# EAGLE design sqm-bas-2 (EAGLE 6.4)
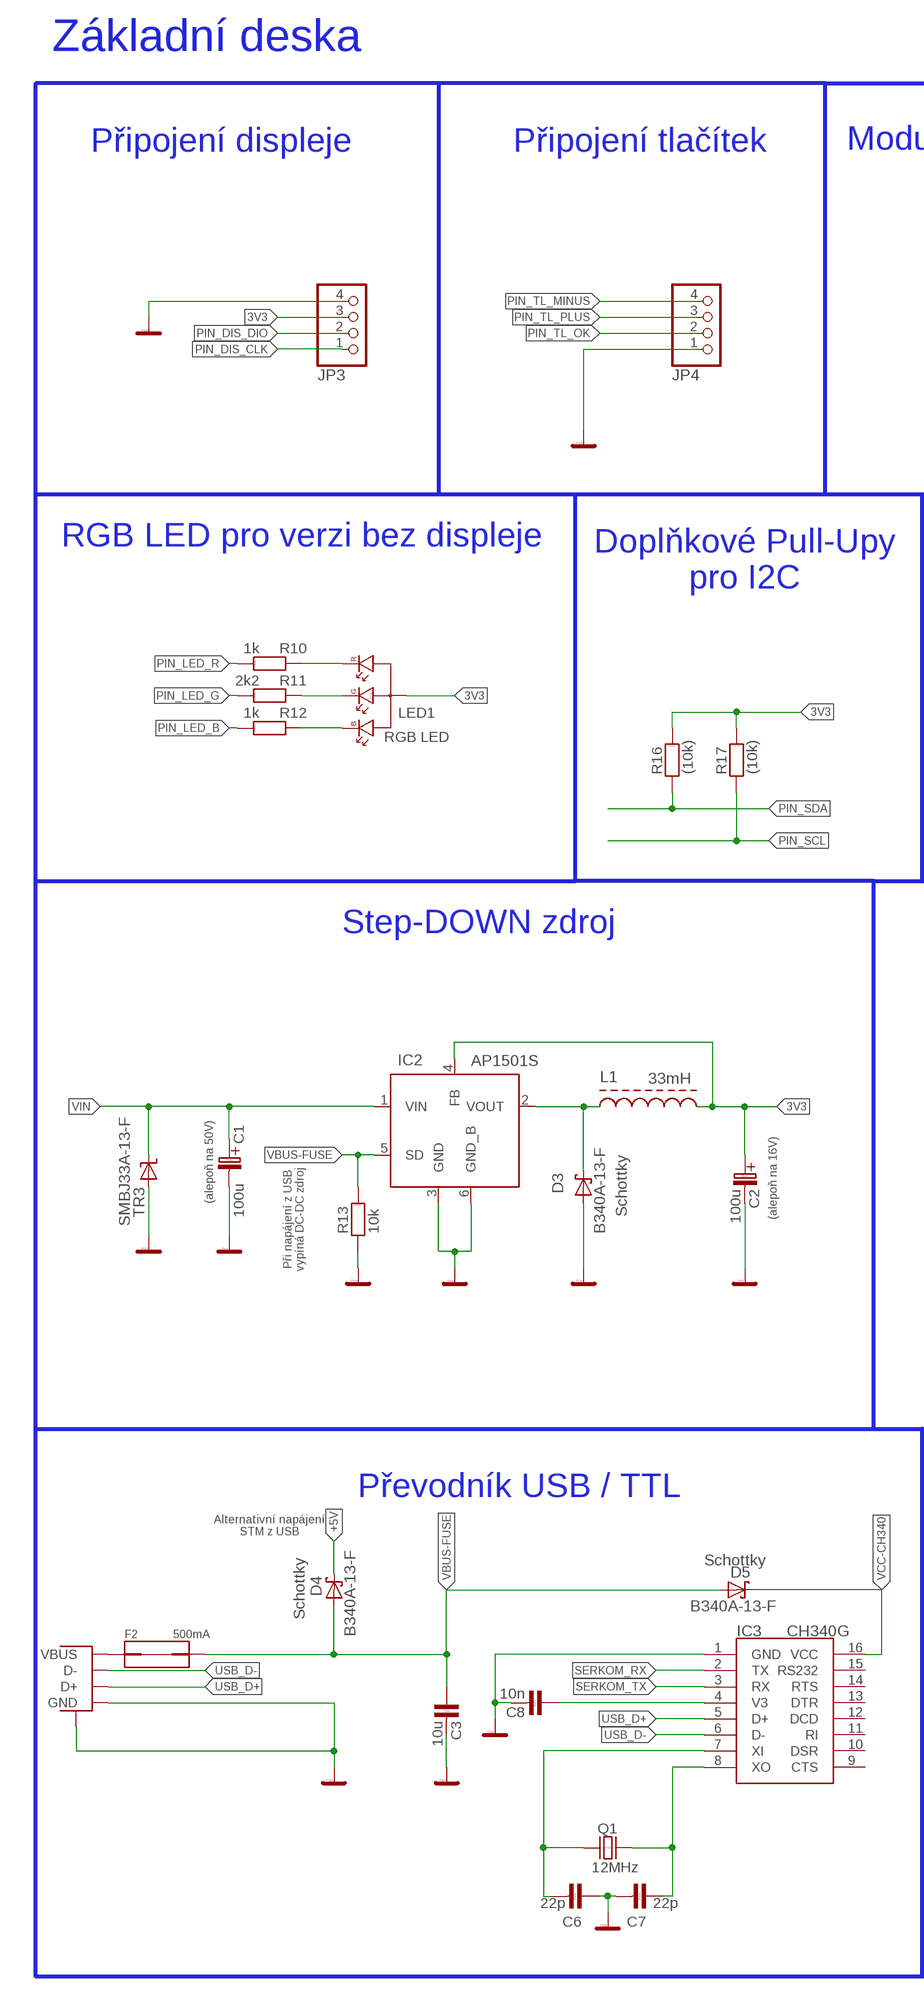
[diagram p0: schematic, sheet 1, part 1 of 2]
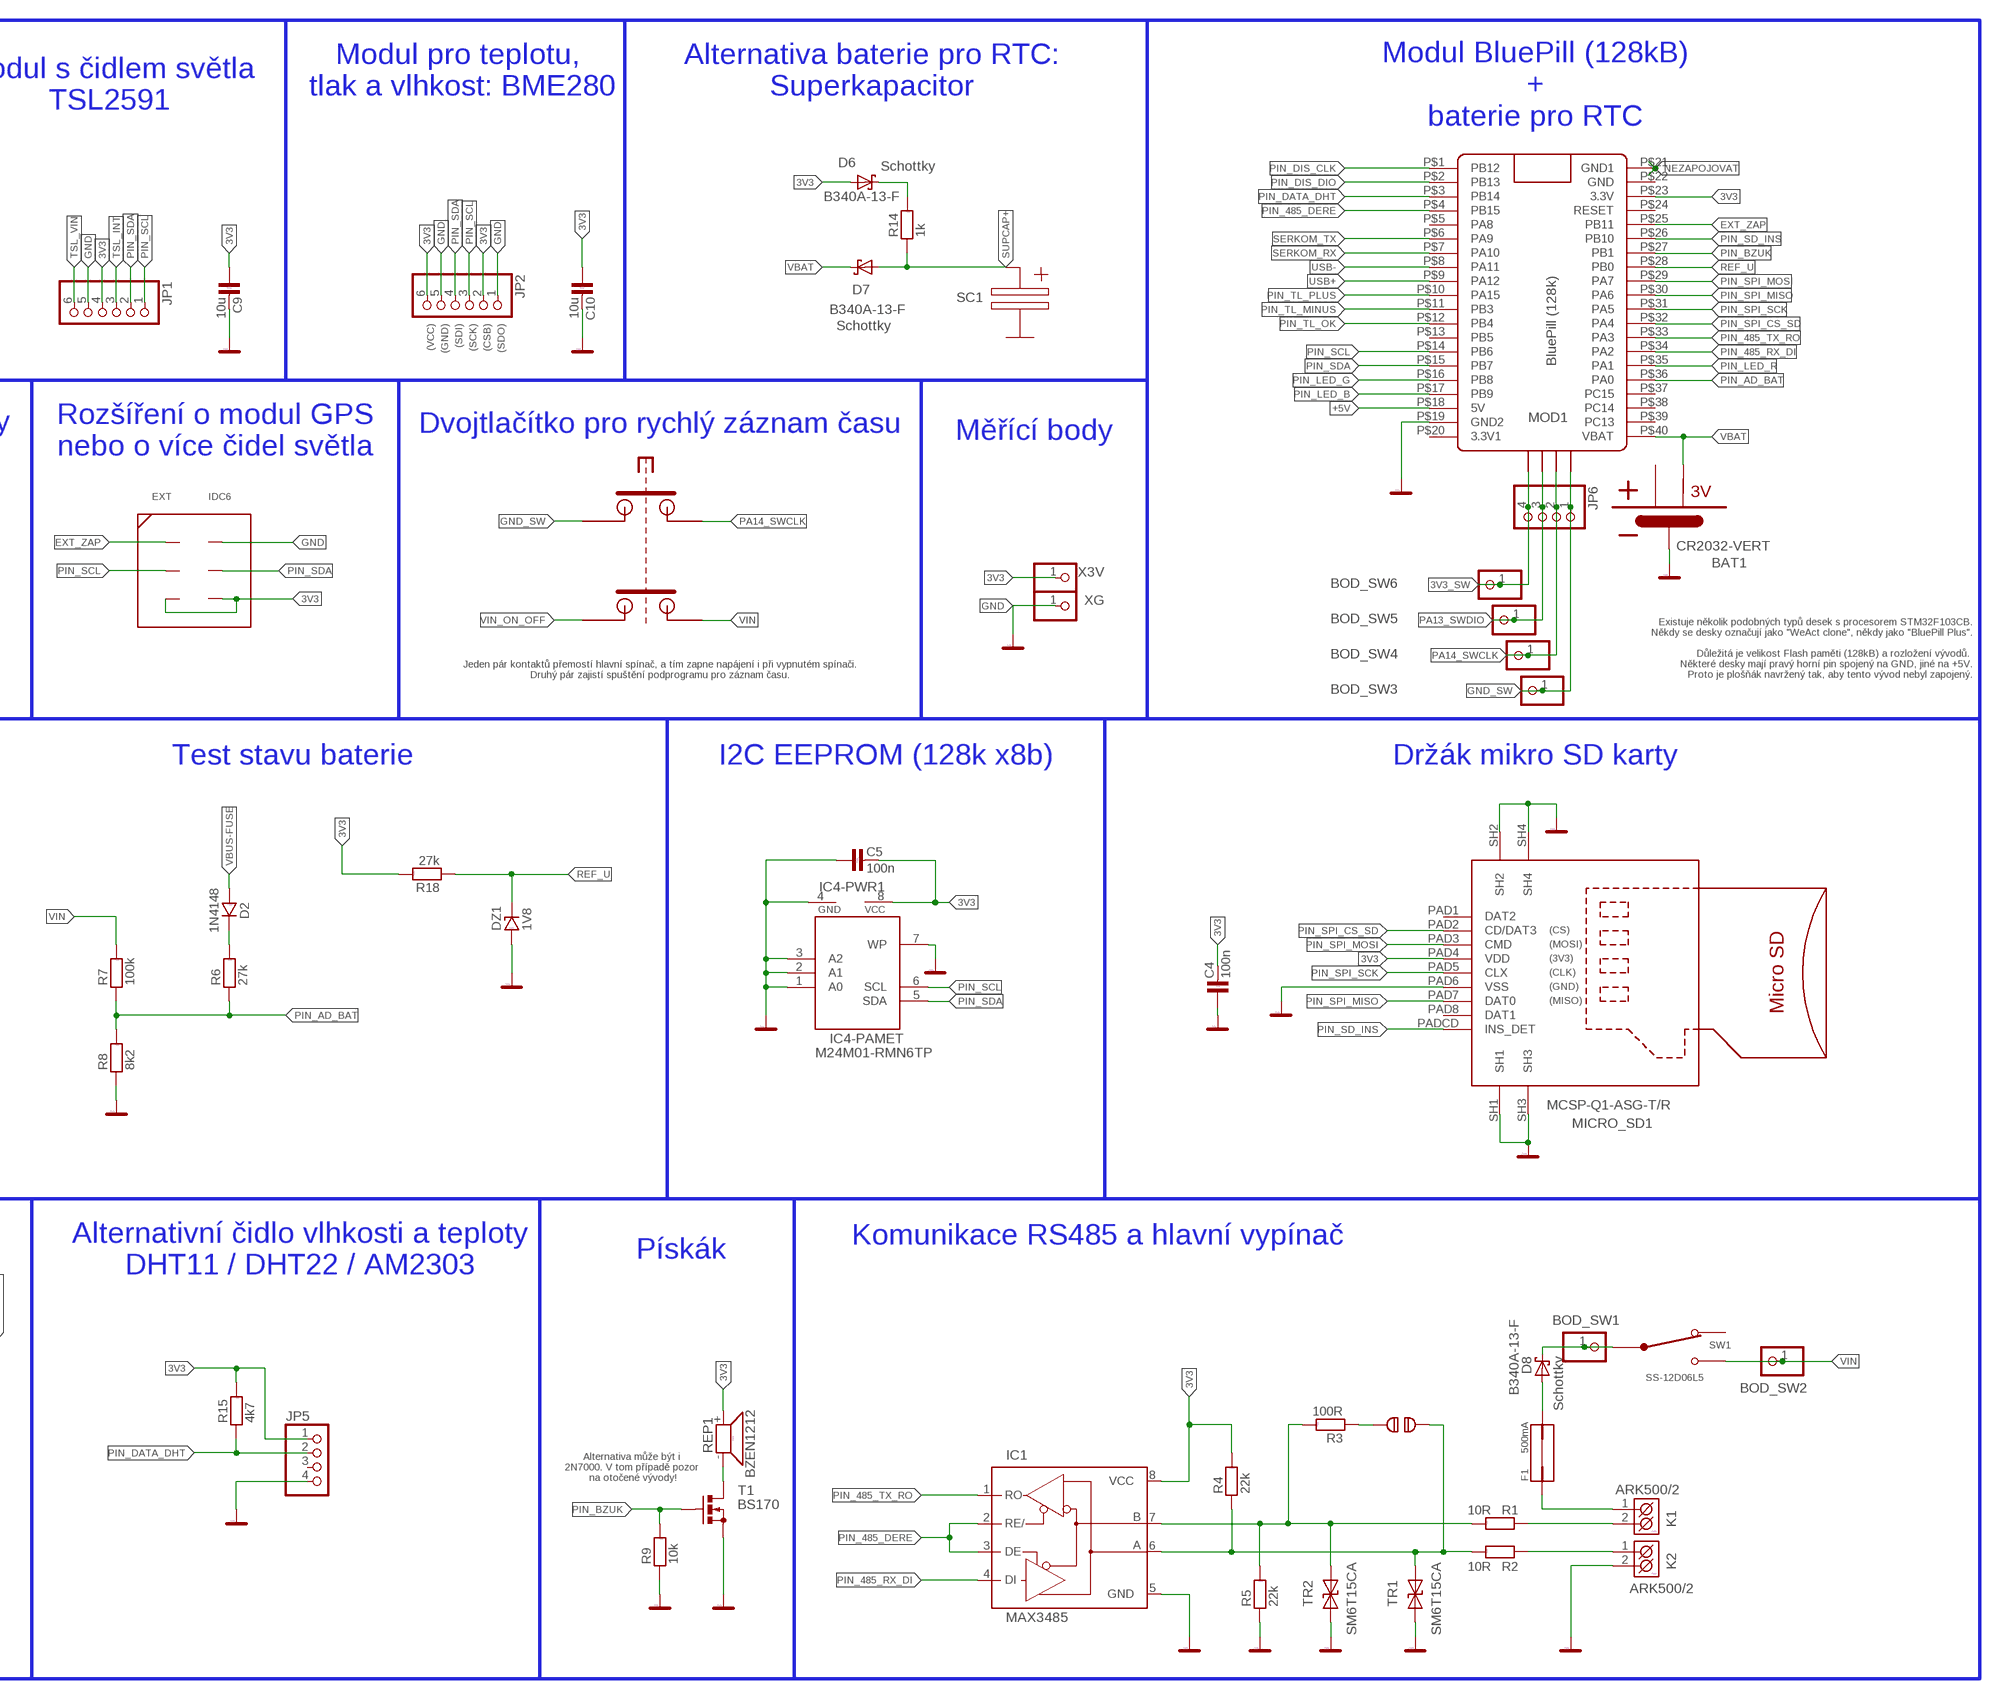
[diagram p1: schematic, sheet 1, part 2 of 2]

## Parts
BAT1  CR2032-VERT  [CR2032-VERT]
BOD_SW1  PINHD-1X1  [1X01]
BOD_SW2  PINHD-1X1  [1X01]
BOD_SW3  PINHD-1X1  [1X01]
BOD_SW4  PINHD-1X1  [1X01]
BOD_SW5  PINHD-1X1  [1X01]
BOD_SW6  PINHD-1X1  [1X01]
C1  100u  C-ELEKTROLYT_3,5  [C-EL_3,5]
C2  100u  C-ELEKTROLYT_3,5  [C-EL_3,5]
C3  10u  C-KERAMIK_SMD_0805  [0805]
C4  100n  C-KERAMIK_SMD_0805  [0805]
C5  100n  C-KERAMIK_SMD_0805  [0805]
C6  22p  C-KERAMIK_SMD_0805  [0805]
C7  22p  C-KERAMIK_SMD_0805  [0805]
C8  10n  C-KERAMIK_SMD_0805  [0805]
C9  10u  C-KERAMIK_SMD_0805  [0805]
C10  10u  C-KERAMIK_SMD_0805  [0805]
D2  1N4148  1N4148_SOD80  [SOD-80]
D3  B340A-13-F  SCHOTTKY-DIODESMD  [SMB]
D4  B340A-13-F  SCHOTTKY-DIODESMD  [SMB]
D5  B340A-13-F  SCHOTTKY-DIODESMD  [SMB]
D6  B340A-13-F  SCHOTTKY-DIODESMD  [SMB]
D7  B340A-13-F  SCHOTTKY-DIODESMD  [SMB]
D8  B340A-13-F  SCHOTTKY-DIODESMD  [SMB]
DZ1  1V8  D-ZENEROVA_0,5W_BZV55C_SMD  [SOD-80]
EXT  IDC6  [IDC6]
F1  500mA  FUSE1812  [FUSE1812]
F2  500mA  FUSE1812  [FUSE1812]
IC1  MAX3485  MAX3468ESA  [SO08]
IC2  AP1501S  [TO263-5]
IC3  CH340G  [SOIC16]
IC4  M24M01-RMN6TP  EEPROM  [SO8]
JP1  PINHD-1X6  [1X06]
JP2  PINHD-1X6  [1X06]
JP3  PINHD-1X4  [1X04]
JP4  PINHD-1X4  [1X04]
JP5  PINHD-1X4  [1X04]
JP6  PINHD-1X4  [1X04]
K1  ARK500/2  [ARK500/2]
K2  ARK500/2  [ARK500/2]
L1  33mH  SMD_INDUCTOR  [SMD_INDUCTOR]
LED1  RGB LED  LED_RGB  [LED_5-RGB]
MICRO_SD1  MCSP-Q1-ASG-T/R  MICRO_SD_MCSP_Q1_A_SG_T_R  [MICRO_SD]
MOD1  BluePill (128k)  BLUE_PILL  [BLUE_PILL]
Q1  12MHz  Q_HC-49U  [HC-49U]
R1  10R  R_1206  [1206]
R2  10R  R_1206  [1206]
R3  100R  R_SMD_0805  [0805]
R4  22k  R_SMD_0805  [0805]
R5  22k  R_SMD_0805  [0805]
R6  27k  R_SMD_0805  [0805]
R7  100k  R_SMD_0805  [0805]
R8  8k2  R_SMD_0805  [0805]
R9  10k  R_SMD_0805  [0805]
R10  1k  R_SMD_0805  [0805]
R11  2k2  R_SMD_0805  [0805]
R12  1k  R_SMD_0805  [0805]
R13  10k  R_SMD_0805  [0805]
R14  1k  R_SMD_0805  [0805]
R15  4k7  R_SMD_0805  [0805]
R16  (10k)  R_SMD_0805  [0805]
R17  (10k)  R_SMD_0805  [0805]
R18  27k  R_SMD_0805  [0805]
REP1  BZEN1212  KPE242  [KPE242]
SJ1  SJ  SOLDERJUMPER  [SJ_2S-NO]
SW1  SS-12D06L5  SLIDE_SW  [SLIDE_SW]
T1  BS170  [SOT54E]
TR1  SM6T15CA  SUPPRESSOR-  [SMBJ]
TR2  SM6T15CA  SUPPRESSOR-  [SMBJ]
TR3  SMBJ33A-13-F  SUPPRESSOR-SMBJ  [SMBJ]
USB1  USBPTH  [USB-B-PTH]
X3V  PINHD-1X1  [1X01]
XG  PINHD-1X1  [1X01]

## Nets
3V3: C2.C+(C_EL+) C4.2 C5.2 C9.1 C10.1 D6.A EXT.P5(PIN5) EXT.P6(PIN6) IC1.8(VCC) IC2.4(FB) IC4.8(-PWR1:VCC) JP1.4 JP2.2 JP2.6 JP3.3 JP5.1 L1.P$2 LED1.2(A) MICRO_SD1.PAD4(VDD) MOD1.P$23(3.3V) R4.2 R15.2 R16.2 R17.2 R18.2 REP1.+ X3V.1
3V3_SW: BOD_SW6.1 JP6.4
+5V: D4.C MOD1.P$18(5V)
BZUK_DRAIN: REP1.- T1.D
CH340-V3: C8.1 IC3.4(V3)
CHARGE: D6.C R14.2
D2-R6: D2.K R6.2
DCDC-SW: D3.C IC2.2(VOUT) L1.P$1
EXT_ZAP: EXT.P1(PIN1) MOD1.P$25(PB11)
GND: BAT1.MINUS C1.C-(C_EL-) C2.C-(C_EL-) C3.2 C4.1 C5.1 C6.1 C7.2 C8.2 C9.2 C10.2 D3.A DZ1.A EXT.P2(PIN2) IC1.5(GND) IC2.3(GND) IC2.6(GND_B) IC3.1(GND) IC4.1(-PAMET:A0) IC4.2(-PAMET:A1) IC4.3(-PAMET:A2) IC4.4(-PWR1:GND) IC4.7(-PAMET:WP) JP1.5 JP2.1 JP2.5 JP3.4 JP4.1 JP5.4 K2.2(K2) MICRO_SD1.PAD6(VSS) MICRO_SD1.SH1 MICRO_SD1.SH2 MICRO_SD1.SH3 MICRO_SD1.SH4 MOD1.P$19(GND2) R5.1 R8.1 R9.1 R13.1 T1.S TR1.A TR2.A TR3.A USB1.GND USB1.P$2(SHIELD) XG.1
GND_SW: BOD_SW3.1 JP6.1
LED_BK: LED1.4(B) R12.1
LED_GK: LED1.3(G) R11.1
LED_RK: LED1.1(R) R10.1
NEZAPOJOVAT: MOD1.P$21(GND1)
PA13_SWDIO: BOD_SW5.1 JP6.3
PA14_SWCLK: BOD_SW4.1 JP6.2
PIN_485_DERE: IC1.2(RE/) IC1.3(DE) MOD1.P$4(PB15)
PIN_485_RX_DI: IC1.4(DI) MOD1.P$34(PA2)
PIN_485_TX_RO: IC1.1(RO) MOD1.P$33(PA3)
PIN_AD_BAT: MOD1.P$36(PA0) R6.1 R7.1 R8.2
PIN_BZUK: MOD1.P$27(PB1) R9.2 T1.G
PIN_DATA_DHT: JP5.2 MOD1.P$3(PB14) R15.1
PIN_DIS_CLK: JP3.1 MOD1.P$1(PB12)
PIN_DIS_DIO: JP3.2 MOD1.P$2(PB13)
PIN_LED_B: MOD1.P$17(PB9) R12.2
PIN_LED_G: MOD1.P$16(PB8) R11.2
PIN_LED_R: MOD1.P$35(PA1) R10.2
PIN_SCL: EXT.P3(PIN3) IC4.6(-PAMET:SCL) JP1.1 JP2.3 MOD1.P$14(PB6) R17.1
PIN_SD_INS: MICRO_SD1.PADCD(INS_DET) MOD1.P$26(PB10)
PIN_SDA: EXT.P4(PIN4) IC4.5(-PAMET:SDA) JP1.2 JP2.4 MOD1.P$15(PB7) R16.1
PIN_SPI_CS_SD: MICRO_SD1.PAD2(CD/DAT3) MOD1.P$32(PA4)
PIN_SPI_MISO: MICRO_SD1.PAD7(DAT0) MOD1.P$30(PA6)
PIN_SPI_MOSI: MICRO_SD1.PAD3(CMD) MOD1.P$29(PA7)
PIN_SPI_SCK: MICRO_SD1.PAD5(CLX) MOD1.P$31(PA5)
PIN_TL_MINUS: JP4.4 MOD1.P$11(PB3)
PIN_TL_OK: JP4.2 MOD1.P$12(PB4)
PIN_TL_PLUS: JP4.3 MOD1.P$10(PA15)
REF_U: DZ1.K MOD1.P$28(PB0) R18.1
RS485-A-IN: K2.1(K1) R2.1
RS485-B-IN: K1.2(K2) R1.1
RS485_TERM: R3.1 SJ1.2
RS_485_A: IC1.6(A) R2.2 R4.1 SJ1.1 TR1.C
RS_485_B: IC1.7(B) R1.2 R3.2 R5.2 TR2.C
SERKOM_RX: IC3.2(TX) MOD1.P$7(PA10)
SERKOM_TX: IC3.3(RX) MOD1.P$6(PA9)
SUPCAP+: D7.A R14.1
TSL_INT: JP1.3
TSL_VIN: JP1.6
UBAT: F1.P$2 K1.1(K1)
USB+: MOD1.P$9(PA12)
USB-: MOD1.P$8(PA11)
USB_D+: IC3.5(D+) USB1.D+
USB_D-: IC3.6(D-) USB1.D-
V-USB-IN: F2.P$2 USB1.VBUS
VBAT: BAT1.PLUS2 D7.C MOD1.P$40(VBAT)
VBUS-FUSE: C3.1 D2.A D4.A D5.A F2.P$1 IC2.5(SD) R13.2
VCC-CH340: D5.C IC3.16(VCC)
VIN: BOD_SW2.1 C1.C+(C_EL+) IC2.1(VIN) R7.2 SW1.PIN_2 TR3.C
VIN_FUSE: D8.A F1.P$1
VIN_ON_OFF: BOD_SW1.1 D8.C SW1.PIN_COM
XI: C6.2 IC3.7(XI) Q1.1
XO: C7.1 IC3.8(XO) Q1.2
Unconnected: BAT1.PLUS1 IC3.9(CTS) IC3.10(DSR) IC3.11(RI) IC3.12(DCD) IC3.13(DTR) IC3.14(RTS) IC3.15(RS232) JP5.3 MICRO_SD1.PAD1(DAT2) MICRO_SD1.PAD8(DAT1) MOD1.P$5(PA8) MOD1.P$13(PB5) MOD1.P$20(3.3V1) MOD1.P$22(GND) MOD1.P$24(RESET) MOD1.P$37(PC15) MOD1.P$38(PC14) MOD1.P$39(PC13) SW1.PIN_1

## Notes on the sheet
- Základní deska
- Připojení displeje | Připojení tlačítek
- Modul pro teplotu, 
  tlak a vlhkost: BME280
- Alternativa baterie pro RTC:
  Superkapacitor
- Modul s čidlem světla
  TSL2591
- Modul BluePill (128kB)
  +
  baterie pro RTC
- Schottky
- SC1
- (VCC) | (GND) | (SDI) | (SCK) | (CSB) | (SDO)
- Schottky
- RGB LED pro verzi bez displeje | Dvojtlačítko pro rychlý záznam času
- Rozšíření o modul GPS
  nebo o více čidel světla
- Měřící body
- Doplňkové Pull-Upy
  pro I2C
- Existuje několik podobných typů desek s procesorem STM32F103CB.
  Někdy se desky označují jako "WeAct clone", někdy jako "BluePill Plus".
  
  Důležitá je velikost Flash paměti (128kB) a rozložení vývodů. 
  Některé desky mají pravý horní pin spojený na GND, jiné na +5V.
  Proto je plošňák navržený tak, aby tento vývod nebyl zapojený.
- Jeden pár kontaktů přemostí hlavní spínač, a tím zapne napájení i při vypnutém spínači.
  Druhý pár zajistí spuštění podprogramu pro záznam času.
- Step-DOWN zdroj | Test stavu baterie | I2C EEPROM (128k x8b) | Držák mikro SD karty
- Schottky
- (alepoň na 50V)
- Při napájení z USB
  vypíná DC-DC zdroj
- (alepoň na 16V)
- Komunikace RS485 a hlavní vypínač
- Převodník USB / TTL
- Alternativní čidlo vlhkosti a teploty
  DHT11 / DHT22 / AM2303
- Pískák
- Alternativní napájení
  STM z USB
- Schottky
- Schottky
- Schottky
- Alternativa může být i
  2N7000. V tom případě pozor
   na otočené vývody!

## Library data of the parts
BAT1 = cr2032-vert:CR2032-VERT: Vertikální držák pro CR2032
BOD_SW1-BOD_SW6 X3V XG = pinhead:PINHD-1X1: PIN HEADER
C1 C2 = #PaJa_30:C-ELEKTROLYT: Kondenzator - elektrolyticky
C3-C10 = #PaJa_30:C-KERAMIK: Kondenzator - keramicky
D2 = #PaJa_30:1N4148: Univerzalni dioda - 0,15A, 75V
D3-D8 = diode:SCHOTTKY-DIODE: Schottky Diode
DZ1 = #PaJa_30:D-ZENEROVA: Zenerova dioda
EXT = idc6:IDC6
F1 F2 = fuse1812:FUSE1812
IC1 = maxim:MAX34*: +5V, Fail-Safe, 40Mbps, Profibus RS-485/RS-422 Transceivers Source: MAX3465-MAX3469.pdf; MPN: MAX3468ESA+T; OC_FARNELL: unknown; OC_NEWARK: 76K6724
IC2 = AP1501:AP1501: AP1501 - Step-Down driver
IC3 = usb-serial:CH340G
IC4 = eeprom:EEPROM: EEPROM
JP1 JP2 = pinhead:PINHD-1X6: PIN HEADER
JP3-JP6 = pinhead:PINHD-1X4: PIN HEADER
K1 K2 = #PaJa_konektory:ARK500/2: Svorkovnice - roztec 5mm - dvojita
L1 = SMD_inductor:SMD_INDUCTOR
LED1 = #PaJa_31:LED_RGB: LED dioda - RGB - trojbarevna - 4 vyvody, spol. Anoda
MICRO_SD1 = micro_SD:MICRO_SD_MCSP_Q1_A_SG_T_R: Micro SD card holder
MOD1 = BluePill:BLUE_PILL
Q1 = #PaJa_30:Q_HC-49U: Krystal - 1MHz - 48MHz
R1 R2 = #PaJa_31:R: Rezistor
R3-R18 = #PaJa_30:R: Rezistor
REP1 = tuk_bzuk_6,6_14:KPE242: Piezo-sirenka - 70dB - 3V az 16V
SJ1 = solderjump:SOLDERJUMPER: Pájecí propojka
SW1 = SLIDE_SW:SLIDE_SW: Posuvny prepinac
T1 = transistor-small-signal:BS170: N-CHANNEL MOS FET
TR1 TR2 = obousmerny_transil:SUPPRESSOR-: Obousmerny transil
TR3 = diode:SUPPRESSOR-: Suppressor diode
USB1 = USB-B:USB: USB Connectors USB-B-PTH is fully proven SKU : PRT-00139 USB-miniB is fully proven SKU : PRT-00587 USB-A-PCB is untested. USB-A-H is C@H proven USB-B-SMT is throughly reviewed, but untested. Needs silkscreen touching up. USB-A-S has not been used/tested USB-MB-H has not been used/tested

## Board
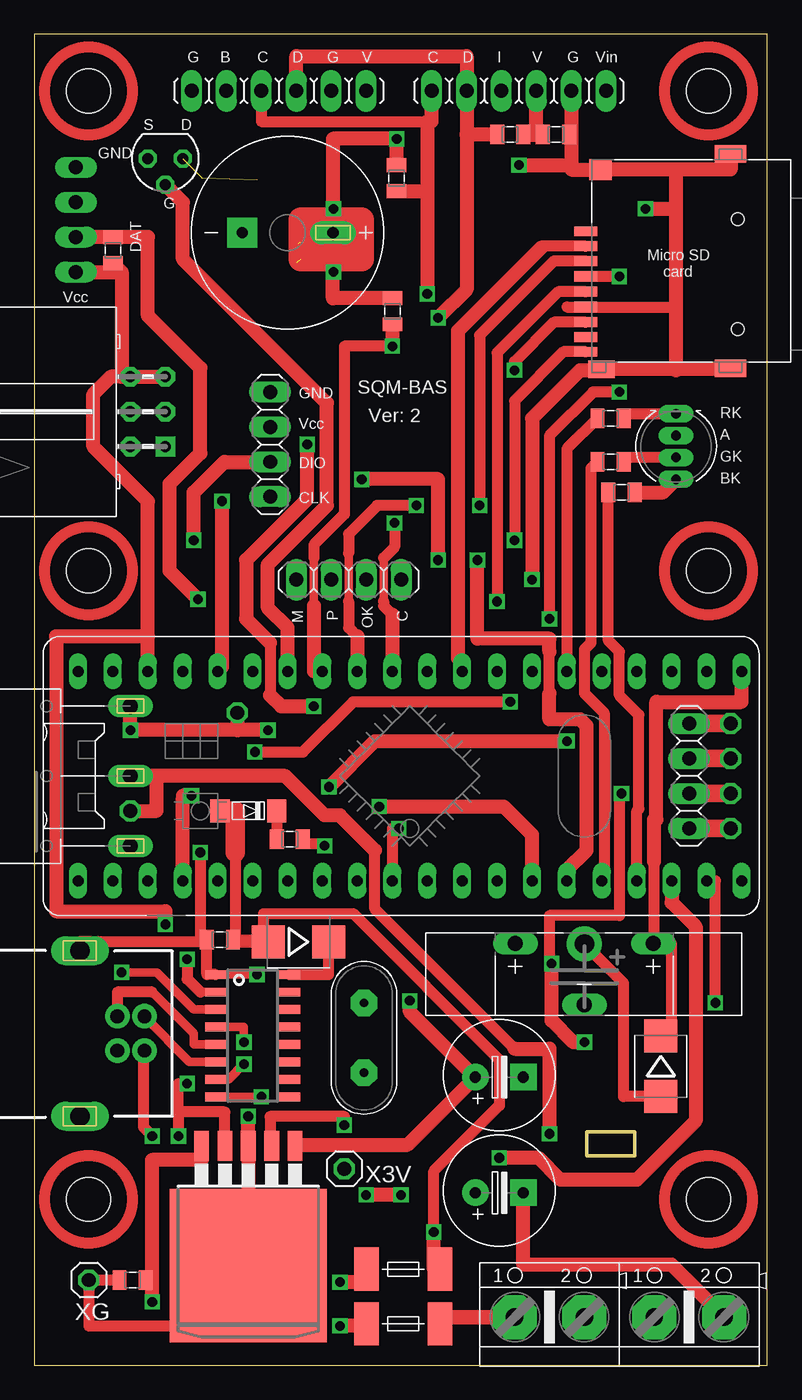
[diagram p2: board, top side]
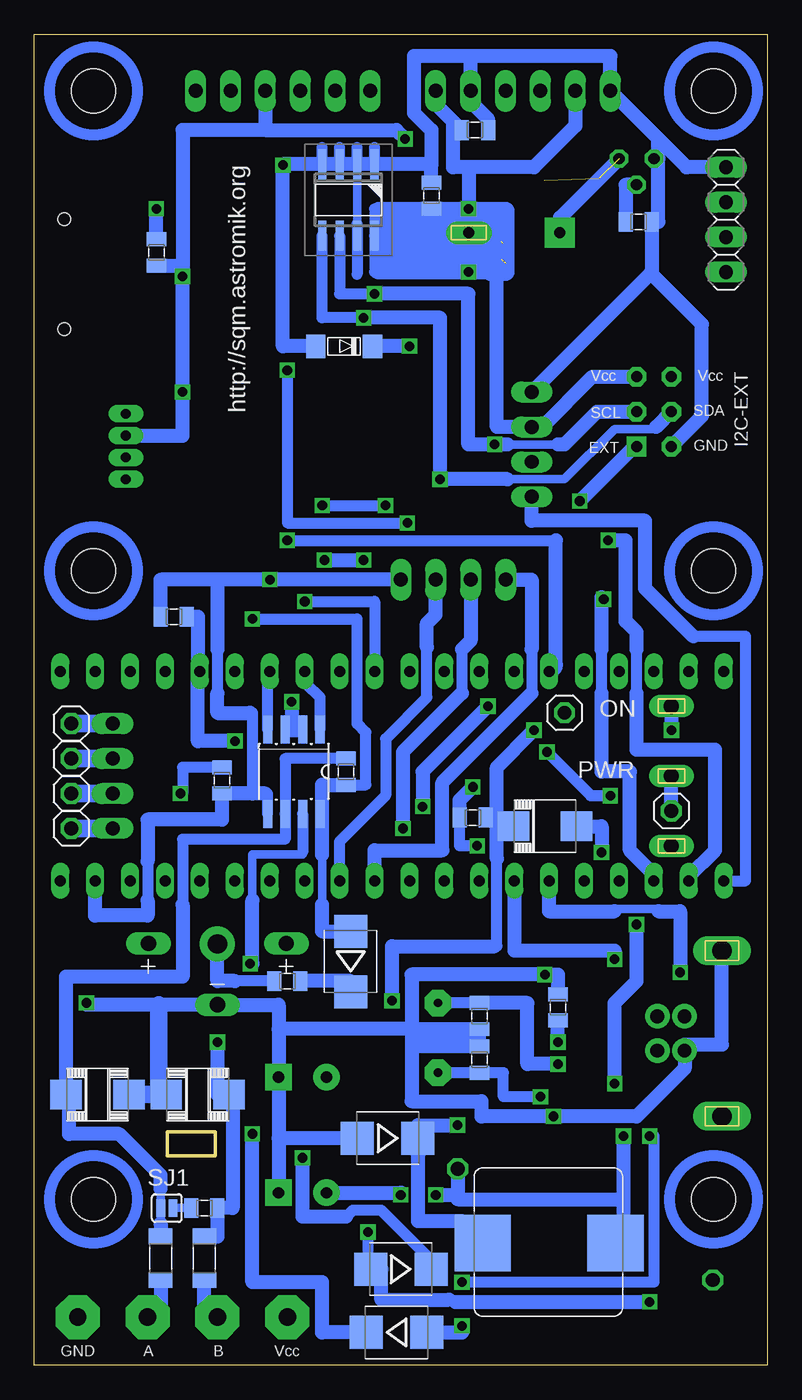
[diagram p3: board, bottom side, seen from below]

Size 53.32 x 96.83 mm. Coordinates in mm from the lower left corner, seen from the top.
Outline: 0,0 53.32,0 53.32,96.83 0,96.83 0,0
Copper layers (1*16): Top 0.035mm / dielectric 1.5mm / Bottom 0.035mm
Design rules "default *": minimum track width 10mil, minimum drill 24mil, track to track 8mil, track to pad 8mil, pad to pad 8mil, via to via 8mil, smd to smd 8mil, copper to edge 40mil, drill to drill 8mil, minimum pad ring 10mil, minimum via ring 8mil, stop-mask expansion 4mil, vias tented up to drill 0mil, thermal gap 10mil
Holes 3.2 mm at 49.02,57.78 3.94,92.71 49.02,92.71 3.94,57.78 3.94,12.06 49.02,12.06
Milling: 4 lines

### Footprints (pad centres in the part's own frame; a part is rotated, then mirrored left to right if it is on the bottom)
CR2032-VERT = drill 1.1 long: MINUS 0,-2.032; PLUS1 -5.016,2.413; PLUS2 5.016,2.413
1X01 = drill 1.016 octagon: 1 0,0
C-EL_3,5 = drill 0.813 pad 1.93: C+ 0,0 | drill 0.813 pad 1.93 square: C- 3.493,0
0805 = smd 1.016 x 1.422: 1 -0.953,0; 2 0.953,0
SOD-80 = smd 1.397 x 1.702: A 1.905,0; K -2.223,0
SMB = smd 2.4 x 2.4: A 2.2,0; C -2.2,0
IDC6 = drill 0.8 pad 1.422 square: P1 -2.54,-2.54 | drill 0.8 pad 1.422 octagon: P2 -2.54,0; P3 0,-2.54; P4 0,0; P5 2.54,-2.54; P6 2.54,0
FUSE1812 = smd 1.778 x 3.15: P$1 -2.667,0; P$2 2.667,0
SO08 = smd 0.66 x 2.032: 1 -1.905,-3.073; 2 -0.635,-3.073; 3 0.635,-3.073; 4 1.905,-3.073; 5 1.905,3.073; 6 0.635,3.073; 7 -0.635,3.073; 8 -1.905,3.073
TO263-5 = smd 1.067 x 2.159: 1 -3.404,-5.791; 2 -1.702,-5.791; 3 0,-5.791; 4 1.702,-5.791; 5 3.404,-5.791 | smd 11.43 x 11.176: 6 0,2.921
SOIC16 = smd 0.635 x 1.524: 1 -4.445,-2.695; 2 -3.175,-2.695; 3 -1.905,-2.695; 4 -0.635,-2.695; 5 0.635,-2.695; 6 1.905,-2.695; 7 3.175,-2.695; 8 4.445,-2.695; 9 4.445,2.695; 10 3.175,2.695; 11 1.905,2.695; 12 0.635,2.695; 13 -0.635,2.695; 14 -1.905,2.695; 15 -3.175,2.695; 16 -4.445,2.695
SO8 = smd 0.6 x 2.2: 1 -1.905,-2.6; 2 -0.635,-2.6; 3 0.635,-2.6; 4 1.905,-2.6; 5 1.905,2.6; 6 0.635,2.6; 7 -0.635,2.6; 8 -1.905,2.6
1X06 = drill 1.016 long: 1 -6.35,0; 2 -3.81,0; 3 -1.27,0; 4 1.27,0; 5 3.81,0; 6 6.35,0
1X04 = drill 1.016 long: 1 -3.81,0; 2 -1.27,0; 3 1.27,0; 4 3.81,0
ARK500/2 = drill 1.27 pad 3.2 octagon: 1 -2.54,0; 2 2.54,0
SMD_INDUCTOR = smd 4.089 x 4.089: P$1 -4.826,0; P$2 4.826,0
LED_5-RGB = drill 0.7 pad 1.27 long: 1 -2.54,0; 2 -0.953,0; 3 0.635,0; 4 2.223,0
MICRO_SD = smd 0.711 x 1.676: PAD1 2.159,7.684; PAD2 1.079,7.684; PAD3 0,7.684; PAD5 -2.223,7.684; PAD7 -4.445,7.684; PAD8 -5.524,7.684; PADCD -6.604,7.684 | smd 0.762 x 1.676: PAD4 -1.111,7.684; PAD6 -3.334,7.684 | smd 1.27 x 1.905: SH1 -7.874,6.54 | smd 1.524 x 1.651: SH2 6.668,6.604 | smd 1.27 x 2.286: SH3 -7.811,-2.857; SH4 7.811,-2.857 | hole 0.9: -4.953,-3.365; 3.048,-3.365
BLUE_PILL = drill 0.8 long: P$1 -7.62,15.24; P$2 -7.62,12.7; P$3 -7.62,10.16; P$4 -7.62,7.62; P$5 -7.62,5.08; P$6 -7.62,2.54; P$7 -7.62,0; P$8 -7.62,-2.54; P$9 -7.62,-5.08; P$10 -7.62,-7.62; P$11 -7.62,-10.16; P$12 -7.62,-12.7; P$13 -7.62,-15.24; P$14 -7.62,-17.78; P$15 -7.62,-20.32; P$16 -7.62,-22.86; P$17 -7.62,-25.4; P$18 -7.62,-27.94; P$19 -7.62,-30.48; P$20 -7.62,-33.02; P$21 7.62,15.24; P$22 7.62,12.7; P$23 7.62,10.16; P$24 7.62,7.62; P$25 7.62,5.08; P$26 7.62,2.54; P$27 7.62,0; P$28 7.62,-2.54; P$29 7.62,-5.08; P$30 7.62,-7.62; P$31 7.62,-10.16; P$32 7.62,-12.7; P$33 7.62,-15.24; P$34 7.62,-17.78; P$35 7.62,-20.32; P$36 7.62,-22.86; P$37 7.62,-25.4; P$38 7.62,-27.94; P$39 7.62,-30.48; P$40 7.62,-33.02
HC-49U = drill 0.61 pad 1.93 octagon: 1 -2.54,0; 2 2.54,0
1206 = smd 1.143 x 1.702: 1 -1.587,0; 2 1.587,0
KPE242 = drill 0.813 pad 1.676 long: + -3.302,0 | drill 0.813 pad 2.184 square: - 3.302,0
SJ_2S-NO = smd 0.635 x 1.27: 1 0,0; 2 0.889,0
SLIDE_SW = drill 1.1 long: PIN_1 -5.08,-7.62; PIN_2 5.08,-7.62; PIN_COM 0,-7.62
SOT54E = drill 0.813 octagon: D -1.27,0; G 0,1.905; S 1.27,0
SMBJ = smd 2.286 x 2.16: A 2.294,0; C -2.284,0
USB-B-PTH = drill 1 pad 1.778: D+ 0,1.25; D- 1.981,1.25; GND 0,-1.25; VBUS 1.981,-1.25 | drill 1.4 long: P$2 -2.718,6.02; SHIELD -2.718,-6.02

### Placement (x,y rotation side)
BAT1  40.01,28.26 0 top
BOD_SW1  6.99,40.32 0 bottom
BOD_SW2  14.76,47.47 0 bottom
BOD_SW3  50.64,46.67 0 bottom
BOD_SW4  50.64,44.13 0 bottom
BOD_SW5  50.64,41.59 0 bottom
BOD_SW6  50.64,39.05 0 bottom
C1  32.07,20.95 0 top
C2  32.07,12.54 0 top
C3  13.49,30.96 180 top
C4  44.45,80.96 270 bottom
C5  24.45,85.09 270 bottom
C6  20.95,25.4 90 bottom
C7  20.95,22.23 90 bottom
C8  15.24,26.04 90 bottom
C9  37.94,89.53 0 top
C10  21.27,89.85 0 bottom
D2  15.4,40.32 180 top
D3  27.62,16.51 180 bottom
D4  26.67,6.99 180 bottom
D5  19.21,30.8 180 top
D6  30.32,29.37 90 bottom
D7  45.56,21.75 270 top
D8  26.99,2.38 0 bottom
DZ1  30.96,74.14 180 bottom
EXT  6.99,69.37 90 top
F1  26.83,3.02 0 top
F2  26.83,6.99 180 top
IC1  34.45,43.18 180 bottom
IC2  15.56,10.16 180 top
IC3  15.88,23.97 270 top
IC4  30.48,84.77 180 bottom
JP1  35.24,92.71 0 top
JP2  17.78,92.71 0 top
JP3  17.14,66.99 90 top
JP4  22.86,57.15 180 top
JP5  3.02,83.34 90 bottom
JP6  47.62,42.86 270 top
K1  37.47,3.49 0 top
K2  47.62,3.49 0 top
L1  15.88,8.89 0 bottom
LED1  46.67,66.67 270 top
MICRO_SD1  47.78,80.33 90 top
MOD1  18.41,42.86 90 top
Q1  23.97,23.81 270 top
R1  40.96,7.78 90 bottom
R2  44.13,7.78 90 bottom
R3  40.96,11.43 0 bottom
R4  30.64,43.18 270 bottom
R5  39.69,42.55 90 bottom
R6  18.57,38.26 180 top
R7  21.43,39.85 0 bottom
R8  43.18,54.45 0 bottom
R9  9.37,83.19 180 bottom
R10  41.91,68.9 180 top
R11  41.91,65.72 180 top
R12  42.7,63.5 180 top
R13  7.14,6.19 0 top
R14  34.92,27.94 0 bottom
R15  5.71,81.12 270 top
R16  34.61,89.53 0 top
R17  26.35,86.36 90 top
R18  26.04,76.68 90 top
REP1  18.41,82.39 180 top
SJ1  44.13,11.43 0 bottom
SW1  -0.64,42.86 90 top
T1  9.53,87.79 180 top
TR1  48.74,19.68 0 bottom
TR2  41.43,19.68 180 bottom
TR3  16.19,39.21 0 bottom
USB1  6.03,24.13 0 top
X3V  22.54,14.29 0 top
XG  3.97,6.19 0 top

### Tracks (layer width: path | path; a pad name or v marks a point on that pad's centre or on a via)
3V3  (via drill 0.7)  (2 unrouted)
  Top 0.813: IC2.4 13.86,18.41 10.48,18.41 | 10.48,18.41 v10.48,16.67 | 10.48,18.41 10.48,20.48 v11.11,20.48 | MICRO_SD1.PAD4 v42.55,79.22 | v42.55,70.8 40.64,70.8 37.47,67.63 v37.47,54.29
  Top 1.016: v26.67,12.38 v24.13,12.38 | MOD1.P$23 8.26,53.02 | 8.26,53.02 8.26,62.87 4.29,66.83 4.29,70.64 5.56,71.91 6.35,71.91 | R16.2 36.51,89.53 | R17.2 v26.35,89.22 21.72,89.22 REP1.+ 21.72,77.63 R18.2 | 8.26,53.02 1.59,53.02 1.59,33.02 9.53,33.02 v9.53,32.07 | EXT.P5 EXT.P6 6.35,71.91 | JP5.1 6.35,79.53 | 6.35,79.53 6.35,71.91 | R15.2 6.35,79.53 | C9.1 36.51,89.53 | 36.51,89.53 JP1.4
  Top 1.778: 21.72,83.34 23.81,83.34 23.81,80.49 19.37,80.49 19.37,82.07 | 19.37,82.07 19.37,83.34 21.72,83.34 | 19.37,82.07 23.5,82.07 | 21.72,83.34 REP1.+
  Bottom 0.406: IC1.8 32.38,40.27 32.38,41.75
  Bottom 0.61: 10.48,8.89 L1.P$2 | 42.55,80.01 v42.55,79.22 | 32.38,33.5 32.38,37.15
  Bottom 0.813: R4.2 29.21,42.23 29.21,46.04 29.84,46.67 29.84,54.29 v37.47,54.29 | C5.2 28.57,84.14 IC4.8 28.57,79.53 28.42,79.53 | 31.91,12.54 C2.C+
  Bottom 1.016: v10.48,16.67 10.48,12.06 | 10.48,12.06 10.48,8.89 | 31.91,12.54 26.67,12.54 v26.67,12.38 | v24.13,12.38 22.54,12.38 | 22.54,12.38 22.54,12.06 10.48,12.06 | v11.11,20.48 11.11,26.35 9.53,27.94 v9.53,32.07 | 28.42,79.53 v21.75,79.53 19.68,79.53 19.68,68.26 JP3.3 16.38,68.26 12.73,71.91 EXT.P5 | JP2.2 13.97,90.17 16.99,87.15 21.72,87.15 | 21.72,87.15 22.86,87.15 22.86,90.49 | JP1.4 36.51,89.85 | 36.51,89.85 42.55,89.85 v42.55,79.22 v42.55,70.8 42.55,67.63 LED1.2 | 36.51,89.85 26.99,89.85 v26.35,89.22 | C4.2 42.55,80.01 | X3V.1 22.54,12.38 | D6.A 32.38,31.57 32.38,33.5 | 32.38,37.15 32.38,41.75 32.38,42.23 R4.2 | C5.2 v21.75,84.14 21.72,84.14 REP1.+ 21.72,87.15 | 22.86,90.49 23.97,91.6 23.97,92.55 JP2.6 | C10.1 22.86,90.49
  Bottom 1.27: 28.26,80.17 19.05,80.17 19.05,83.98 27.94,83.98 | 27.94,83.98 27.94,81.12 24.92,81.12 24.92,83.03 26.99,83.03 26.99,81.76 25.88,81.76 25.88,82.71 | 19.21,81.6 19.05,81.6 19.05,79.53 20.16,79.53 20.16,80.33 | 25.88,81.6 28.26,81.6 28.26,83.98 27.94,83.98
  Bottom 1.778: 21.72,80.49 19.37,80.49 19.37,81.76 | 23.81,81.76 23.81,80.49 21.72,80.49 | 23.81,81.76 23.81,83.34 19.37,83.34 19.37,81.76 | 19.37,81.76 23.81,81.76 | 21.72,80.49 REP1.+
3V3_SW
  Top 1.27: JP6.4 BOD_SW6.1
  Bottom 1.27: JP6.4 BOD_SW6.1
+5V  (via drill 0.7)
  Top 1.016: v33.81,15.08 36.67,15.08 38.26,13.49 43.81,13.49 48.1,17.78 48.1,31.91 46.35,33.66 MOD1.P$18
  Bottom 0.813: 24.47,7.3 24.61,7.3 24.61,7.78 28.1,11.27 30.16,11.27 30.64,10.79
  Bottom 1.016: D4.C 24.47,7.3 | 30.64,10.79 33.81,10.79 v33.81,15.08
BZUK_DRAIN  (2 unrouted)
  Bottom 1.016: T1.D 15.08,83.5 15.08,82.39 REP1.-
CH340-V3  (via drill 0.7)
  Top 0.61: IC3.4 15.24,24.61 v15.24,23.5
  Bottom 1.016: v15.24,23.5 C8.1
CHARGE
  Bottom 0.813: D6.C 30.32,27.94
  Bottom 1.016: 30.32,27.94 R14.2
D2-R6
  Top 0.813: D2.K R6.2
DCDC-SW  (via drill 0.7)
  Top 0.61: 17.14,15.95 IC2.2
  Top 0.813: 17.14,15.95 17.14,18.1 22.54,18.1 v22.54,17.46
  Bottom 0.61: L1.P$1 22.23,8.89 22.23,10.48
  Bottom 1.016: 22.23,10.48 25.4,10.48 25.4,15.24 | v22.54,17.46 25.4,17.46 25.4,15.24 | 25.4,15.24 25.42,15.26 D3.C
EXT_ZAP  (via drill 0.7)
  Top 1.016: MOD1.P$25 13.65,50.8 v13.65,62.87
  Bottom 1.016: v13.65,62.87 9.68,66.83 EXT.P1
GND  (via drill 0.7)
  Top 0.61: IC3.1 v16.19,28.42 | 39.69,87 MICRO_SD1.SH2 | 39.05,87.31 39.05,87 | MICRO_SD1.SH3 50.64,72.45 | 39.69,72.39 46.67,72.39 | 46.51,76.99 46.67,77.15
  Top 0.813: IC3.1 12.54,28.42 12.54,30.8 12.06,30.8 | 12.06,30.8 3.33,30.8 3.33,30.15 USB1.P$2 | IC2.6 15.56,2.86 3.97,2.86 XG.1 R13.1 | 38.73,76.99 MICRO_SD1.PAD6 46.51,76.99 | v12.06,37.31 12.06,30.8 | v49.53,26.35 49.53,35.24 MOD1.P$19
  Top 1.016: IC2.6 IC2.3 v15.56,18.1 | MICRO_SD1.SH4 50.64,87 46.67,87 | 46.67,87 MICRO_SD1.SH2 39.05,87 | JP1.5 39.05,89.53 | 50.64,72.45 MICRO_SD1.SH1 | 46.67,72.39 46.67,77.15 46.67,84.14 | 46.67,84.14 46.67,87 | v35.24,87.31 39.05,87.31 39.05,89.53 | v36.2,57.15 36.2,68.9 39.69,72.39 41.24,72.39 MICRO_SD1.SH1 | v44.45,84.14 46.67,84.14 | C2.C- 35.56,7.3 46.35,7.3 K2.2 | C9.2 39.05,89.53 | C3.2 12.54,30.8 | MICRO_SD1.SH1 41.27,72.45 41.27,72.55
  Bottom 0.61: 3.17,30.15 USB1.P$2 | 11.11,92.71 JP2.1 | IC4.7 29.84,83.03 IC4.2 | 35.24,87.37 v35.24,87.31
  Bottom 0.813: IC1.5 36.35,41.59 36.51,41.59 | 45.09,36.67 45.09,33.81 | 40.01,52.7 40.01,52.07 40.01,48.9 | 37.62,47.47 37.47,47.47 37.47,41.59 | 29.84,83.03 29.84,79.38 | IC4.1 28.57,88.58 | IC4.3 31.11,88.58 | IC4.4 32.38,88.58 | IC4.2 29.84,88.58
  Bottom 1.016: 35.56,16.51 C1.C- 35.56,24.45 | 35.56,16.51 C2.C- | 25.88,24.45 25.88,28.42 v16.19,28.42 15.24,28.42 C8.2 | 25.88,24.45 C6.1 C7.2 21.27,23.18 | 35.56,24.45 35.56,26.23 BAT1.MINUS 44.29,26.23 49.53,26.23 v49.53,26.35 | D3.A 35.56,16.51 | 25.88,24.45 35.56,24.45 | 36.51,41.59 37.47,41.59 R5.1 39.69,39.69 45.09,39.69 45.09,36.67 | 45.09,33.81 45.09,32.7 48.9,32.7 MOD1.P$19 | JP4.1 v36.2,57.15 40.01,57.15 | 37.62,47.47 40.01,47.47 40.01,48.9 | 21.59,95.25 11.43,95.25 JP2.1 7.94,89.22 | 21.59,95.25 JP2.5 21.59,91.92 20.32,90.65 C10.2 | 21.59,95.25 25.72,95.25 25.72,91.12 24.45,89.85 24.45,87.37 | 24.45,87.37 IC4.1 IC4.2 IC4.3 IC4.4 35.24,87.37 | C4.1 v44.45,84.14 | 40.01,57.15 40.01,52.07 | C5.1 24.45,87.37 | 3.17,30.01 USB1.P$2 3.31,23.34 6.03,23.34 USB1.GND 6.03,21.59 9.53,18.1 v15.56,18.1 20.8,18.1 20.8,19.21 25.88,19.21 25.88,24.29 | TR3.A 12.06,39.21 v12.06,37.31 | 8.49,79.45 8.41,79.53 R9.1 7.94,83.19 7.94,87.79 | 8.49,79.45 JP3.4 | EXT.P2 4.76,69.06 4.76,75.72 8.49,79.45 | JP5.4 5.87,87.15 7.94,89.22 | T1.S 7.94,87.79 | 7.94,87.79 7.94,89.22 | 25.56,23.81 21.27,23.81 21.27,23.18 | 21.27,23.18 25.72,23.18 | DZ1.A 35.24,74.14 v35.24,87.31 | 40.01,57.15 44.13,57.15 R8.1
  Bottom 1.27: TR1.A 44.29,19.68 | 44.29,19.68 44.29,26.23 | TR2.A 44.29,19.68
GND_SW
  Top 1.27: JP6.1 BOD_SW3.1
  Bottom 1.27: JP6.1 BOD_SW3.1
LED_BK
  Top 0.61: LED1.4 46.35,64.45
  Top 1.016: R12.1 45.72,63.5 LED1.4
LED_GK
  Top 0.61: 42.86,66.04 R11.1
  Top 0.813: LED1.3 42.86,66.04
LED_RK
  Top 0.61: R10.1 42.86,69.22
  Top 0.813: 42.86,69.22 LED1.1
PA13_SWDIO
  Top 1.27: JP6.3 BOD_SW5.1
  Bottom 1.27: JP6.3 BOD_SW5.1
PA14_SWCLK
  Top 1.27: JP6.2 BOD_SW4.1
  Bottom 1.27: JP6.2 BOD_SW4.1
PIN_485_DERE  (via drill 0.7)
  Top 0.813: v34.61,48.26 23.18,48.26 19.53,44.61 v16.03,44.61 | 10.79,41.43 10.79,41.27
  Top 1.016: v11.43,41.43 10.79,41.43 | MOD1.P$4 10.79,41.27
  Bottom 0.61: IC1.3 IC1.2 34.92,46.25
  Bottom 0.813: 34.92,46.25 34.92,46.2 34.61,46.2 | 34.61,48.1 v34.61,48.26 | v16.03,44.61 12.86,41.43 v11.43,41.43
  Bottom 1.016: 34.61,48.1 34.61,46.35 34.61,46.2 34.29,46.2
PIN_485_RX_DI
  Bottom 0.813: IC1.4 36.35,50.32 MOD1.P$34
PIN_485_TX_RO
  Bottom 0.813: IC1.1 32.54,48.58 33.5,49.53 33.5,50.32 MOD1.P$33
PIN_AD_BAT  (via drill 0.7)
  Top 0.813: R6.1 19.53,37.94 21.11,37.94 v21.11,37.78
  Top 1.016: v21.43,42.07 24.77,45.4 v38.73,45.4
  Bottom 0.813: v21.11,37.78 22.38,37.78 R7.1
  Bottom 1.016: R7.1 22.38,41.12 v21.43,42.07 | v38.73,45.4 41.43,45.4 41.43,50.48 | MOD1.P$36 41.43,50.48 | R8.2 41.43,54.45 41.43,50.48
PIN_BZUK
  Top 1.016: MOD1.P$27 18.41,53.66 16.99,55.09 16.99,58.26 21.27,62.55 21.27,70.01 10.79,80.49 10.79,84.61 T1.G
  Bottom 1.016: T1.G 10.32,85.88 R9.2
PIN_DATA_DHT  (via drill 0.7)
  Top 1.016: v11.91,55.72 9.84,57.78 9.84,64.14 12.06,66.36 12.06,72.55 8.26,76.36 8.26,82.07 R15.1 JP5.2
  Bottom 0.813: 12.06,48.9 12.06,52.07
  Bottom 1.016: 12.06,48.9 12.06,43.18 10,43.18 10,37.47 8.26,35.72 MOD1.P$3 | 12.06,52.07 12.06,55.88 v11.91,55.72
PIN_DIS_CLK
  Bottom 0.813: MOD1.P$1 1.59,35.24 1.59,53.02 5.4,53.02
  Bottom 1.016: 5.4,53.02 8.89,56.52 8.89,61.44 17.14,61.44 JP3.1
PIN_DIS_DIO  (via drill 0.7)
  Top 1.016: v11.59,60.01 11.59,63.5 13.81,65.72 JP3.2
  Bottom 0.813: MOD1.P$2 5.71,35.56 | 9.53,48.9 9.53,52.07
  Bottom 1.016: 5.71,35.56 3.81,37.47 3.81,44.77 9.53,44.77 9.53,48.9 | 9.53,52.07 9.53,53.34 10.32,54.13 10.32,60.01 v11.59,60.01
PIN_LED_B
  Top 0.813: MOD1.P$17 43.81,40.32 43.97,40.48 43.97,47.31 42.55,48.74 42.55,51.91 41.75,52.7 R12.2
PIN_LED_G
  Top 0.813: R11.2 40.48,65.25 40.48,52.55 40.01,52.07 40.01,48.9 41.43,47.47 41.43,35.24 MOD1.P$16
PIN_LED_R
  Top 0.813: R10.2 38.73,66.67 MOD1.P$35
PIN_SCL  (via drill 0.7)
  Top 0.61: 28.57,90.49 28.89,90.49
  Top 0.813: JP2.3 16.51,90.49 28.57,90.49 | 17.14,52.55 17.14,48.74
  Top 1.016: 28.89,90.49 JP1.1 | 28.57,90.49 28.57,85.41 | 28.57,85.41 v28.57,77.95 | R17.1 28.57,85.41 | 17.14,52.55 15.4,54.29 15.4,58.58 19.84,63.02 v19.84,66.99 | MOD1.P$14 36.2,38.58 34.13,40.64 v25.08,40.64 | v20.32,47.94 17.94,47.94 17.14,48.74
  Bottom 0.61: 15.24,66.99 18.89,66.99
  Bottom 0.813: IC4.6 31.11,77.95 v28.57,77.95
  Bottom 1.016: 18.89,66.99 v19.84,66.99 21.75,66.99 21.75,77.95 v28.57,77.95 | v20.32,47.94 25.08,43.18 v25.08,40.64 | EXT.P3 12.38,69.37 14.76,66.99 15.24,66.99
PIN_SD_INS  (via drill 0.7)
  Top 0.813: MICRO_SD1.PADCD 38.48,73.72 34.92,70.17 v34.92,60.01
  Bottom 0.813: v34.92,60.01 15.4,60.01
  Bottom 1.016: MOD1.P$26 arc-90 15.4,50.96 15.4,60.01
PIN_SDA  (via drill 0.7)
  Top 0.813: 37.47,48.9 37.47,51.91
  Top 1.016: JP2.4 19.05,95.25 31.43,95.25 JP1.2 31.43,89.53 | 31.43,89.53 31.43,78.26 v29.37,76.2 | R16.1 31.43,89.53 | MOD1.P$15 38.73,36.04 40.16,37.47 40.16,46.51 39.69,46.99 37.47,46.99 37.47,48.9 | 37.47,51.91 37.47,52.86 32.23,52.86 v32.23,58.58 | v29.37,58.58 29.37,64.45 v23.81,64.45
  Bottom 0.61: 18.89,64.45 14.76,64.45 11.11,68.1 8.26,68.1 8.1,68.26
  Bottom 0.813: v29.37,76.2 32.38,76.2 IC4.5
  Bottom 1.016: 18.89,64.45 v23.81,64.45 23.81,76.2 v29.37,76.2 | v32.23,58.58 v29.37,58.58 | EXT.P4 8.1,68.26
PIN_SPI_CS_SD
  Top 0.61: 36.83,81.41 36.83,81.28
  Top 0.813: MICRO_SD1.PAD2 36.83,81.41
  Top 1.016: MOD1.P$32 31.11,51.12 30.8,51.44 30.8,75.25 36.83,81.28
PIN_SPI_MISO  (via drill 0.7)
  Top 0.61: 25.4,58.74 25.4,55.56
  Top 0.813: MICRO_SD1.PAD7 37.78,75.88 34.92,73.03 v34.92,72.39 | v26.19,61.28 26.19,59.53 25.4,58.74 | 25.4,55.56 25.4,55.24 26.04,54.61
  Top 1.016: 26.04,54.61 MOD1.P$30
  Bottom 0.813: v34.92,72.39 34.92,61.28 v26.19,61.28
PIN_SPI_MOSI  (via drill 0.7)
  Top 0.61: 22.86,59.05 22.86,55.56
  Top 0.813: MICRO_SD1.PAD3 37.78,80.33 32.38,74.93 v32.38,62.55 | v27.78,62.55 24.92,62.55 22.86,60.48 22.86,59.05 | 22.86,55.56 22.86,53.66 23.5,53.02
  Top 1.016: 23.5,53.02 MOD1.P$29
  Bottom 0.813: v32.38,62.55 v27.78,62.55
PIN_SPI_SCK  (via drill 0.7)
  Top 0.813: MICRO_SD1.PAD5 38.1,78.11 33.66,73.66 v33.66,55.56
  Bottom 0.813: v33.66,55.56 28.57,55.56 MOD1.P$31
PIN_TL_MINUS
  Bottom 0.813: 17.14,52.07 17.14,48.9
  Bottom 1.016: JP4.4 17.14,57.15 17.14,52.07 | MOD1.P$11 28.57,37.47 23.65,37.47 23.65,42.39 17.14,48.9
PIN_TL_OK
  Bottom 0.813: MOD1.P$12 31.11,38.1 27.78,41.43 27.78,45.56 24.77,48.58 24.77,52.23
  Bottom 1.016: 24.77,52.23 24.77,53.98 24.13,54.61 JP4.2
PIN_TL_PLUS  (via drill 0.7)
  Top 0.813: v26.51,39.05 26.04,39.05 MOD1.P$10
  Bottom 0.813: 22.23,52.07 22.23,48.9
  Bottom 1.016: JP4.3 21.59,52.7 22.23,52.07 | 22.23,48.9 26.51,44.61 v26.51,39.05
REF_U  (via drill 0.7)
  Top 0.61: 20.32,58.74 20.32,55.24
  Top 0.813: v26.04,74.14 22.54,74.14 22.54,61.91 20.32,59.69 20.32,58.74
  Top 1.016: R18.1 v26.04,74.14 | 20.32,55.24 20.32,50.48 MOD1.P$28
  Bottom 1.016: v26.04,74.14 DZ1.K
RS485-A-IN
  Bottom 1.016: R2.1 44.13,3.49 K2.1
RS485-B-IN
  Bottom 0.61: 40.96,3.49 40.96,3.81
  Bottom 1.016: K1.2 40.96,3.49 | 40.96,3.81 R1.1
RS485_TERM
  Bottom 0.61: SJ1.2 R3.1
RS_485_A
  Bottom 0.61: 44.13,12.86 SJ1.1 44.13,10.32
  Bottom 0.813: 42.55,33.5 42.55,38.26 35.08,38.26 IC1.6 35.08,44.13 R4.1
  Bottom 1.016: 44.13,10.32 R2.2 | 44.13,12.86 44.13,13.81 47.15,16.83 50.8,16.83 50.8,19.68 TR1.C 51.02,28.26 42.55,28.26 42.55,33.5
RS_485_B  (via drill 0.7)
  Top 0.813: v42.7,41.59 42.55,41.59 42.55,32.7 37.47,32.7 37.47,29.21 v37.62,29.21
  Top 1.016: v40.01,23.5 39.21,23.5 37.62,25.08 v37.62,29.21
  Bottom 0.61: 33.81,37.31 33.81,37.15 37.47,37.15 37.47,33.81 37.47,32.86
  Bottom 0.813: IC1.7 33.81,37.31 | R5.2 42.55,43.5 42.55,41.59 v42.7,41.59
  Bottom 1.016: R1.2 40.01,9.37 R3.2 38.89,11.43 38.89,19.68 TR2.C 40.01,19.68 v40.01,23.5 | v37.62,29.21 37.47,29.21 37.47,33.81
SERKOM_RX  (via drill 0.7)
  Top 0.61: IC3.2 12.06,27.15
  Top 0.813: 12.06,27.15 11.11,28.1 v11.11,29.53
  Bottom 1.016: MOD1.P$7 18.41,30.16 11.11,30.16 v11.11,29.53
SERKOM_TX  (via drill 0.7)
  Top 0.61: IC3.3 11.59,25.88 8.89,28.57 v6.35,28.57
  Bottom 0.61: 11.11,33.02 11.11,33.18 7.94,33.18 7.94,33.02
  Bottom 1.016: 11.11,33.02 15.88,33.02 MOD1.P$6 | 7.94,33.02 6.35,33.02 v6.35,28.57
SUPCAP+  (via drill 1.4 pad 2.54)
  Top 0.813: D7.A 42.86,19.55 42.86,27.78 v40.01,30.64
  Bottom 0.813: R14.1 38.73,27.94
  Bottom 1.016: 38.73,27.94 40.01,27.94 v40.01,30.64
UBAT
  Top 0.813: 29.19,3.48 29.21,3.49
  Top 1.016: K1.1 29.53,3.49 | 29.21,3.49 29.53,3.49 | 29.53,3.49 29.53,3.65 | K1.1 35.08,3.49 | K1.1 31.43,3.49 | F1.P$2 29.5,3.49 K1.1
USB_D+
  Top 0.61: 8.57,27.15 11.59,24.13 11.59,23.34 IC3.5
  Top 0.813: 8.57,27.15 6.03,27.15 USB1.D+
USB_D-
  Top 0.61: IC3.6 11.27,22.07 8.01,25.32 USB1.D-
V-USB-IN  (via drill 0.7)
  Top 0.813: v8.57,16.67 7.94,17.3 7.94,22.8 USB1.VBUS
  Top 1.016: 24.16,6.03 v22.23,6.03 | 24.46,6.03 24.16,6.03 | 24.16,6.03 F2.P$2
  Bottom 0.813: v22.23,6.03 8.26,6.03 8.26,16.67 v8.57,16.67
VBAT
  Top 0.813: D7.C 46.35,23.95 46.35,30.67 BAT1.PLUS2 | 45.09,30.64 45.09,36.67
  Top 1.016: BAT1.PLUS2 45.02,30.64 45.09,30.64 | 45.09,36.67 45.09,39.69 45.24,39.69 45.24,48.26 51.44,48.26 MOD1.P$40
VBUS-FUSE  (via drill 0.7)
  Top 0.61: IC2.5 12.15,15.56
  Top 0.813: 29.03,9.21 29.03,7.62 | 29.03,7.62 29.03,6.83 | 14.61,30.96 16.67,30.96 16.67,32.86 23.18,32.86 33.81,22.23 33.81,18.89 29.05,14.13 v29.05,9.68 29.05,7.62 29.03,7.62 | D5.A 14.45,30.8 C3.1 14.61,30.96 | R13.2 8.57,6.19 v8.57,4.6 | 14.61,37.31 14.61,30.96
  Top 1.016: 12.15,15.56 12.15,14.92 8.57,14.92 v8.57,4.6 | F2.P$1 29.05,6.99 v29.05,9.68
  Top 1.422: D2.A 14.61,40.32 14.61,37.31
  Bottom 0.406: 22.7,4.6 22.7,4.76
  Bottom 0.61: 23.18,4.76 22.7,4.76
  Bottom 0.813: D4.A 29.05,6.99 v29.05,9.68
  Bottom 1.016: 23.18,4.76 28.08,4.76 28.08,6.99 D4.A | 22.7,4.6 v8.57,4.6
VCC-CH340
  Top 0.813: IC3.16 21.41,28.42 D5.C
VIN  (via drill 0.7)
  Top 1.016: v16.99,46.2 14.76,46.2 | 14.76,46.2 v6.99,46.2 SW1.PIN_2 | IC2.1 18.96,16.03 27.15,16.03 C1.C+ 27.3,25.72 v27.3,26.51 | BOD_SW2.1 14.76,46.2
  Bottom 0.813: 19.84,30.48 19.68,30.48 19.68,36.83
  Bottom 1.016: v27.3,26.51 27.3,30.48 19.84,30.48 | 19.68,36.83 19.68,39.21 | 19.68,39.85 19.68,43.5 v16.99,46.2 | R7.2 19.68,39.85 | 19.68,39.85 19.68,39.21 | TR3.C 19.68,39.21 | SW1.PIN_2 v6.99,46.2
VIN_FUSE  (via drill 0.7)
  Top 1.016: F1.P$1 24.16,2.86 v22.23,2.86
  Bottom 1.016: D8.A 22.23,2.38 v22.23,2.86
VIN_ON_OFF  (via drill 0.7)
  Top 0.813: 24.77,37.47 24.77,33.18 34.92,23.02
  Top 1.016: 34.92,23.02 37.47,23.02 v37.47,16.83 | 8.89,42.86 18.26,42.86 21.11,40.01 22.23,40.01 24.77,37.47 | 8.89,42.86 SW1.PIN_COM | BOD_SW1.1 8.89,40.32 8.89,42.86
  Bottom 1.016: v37.47,16.83 37.47,6.03 32.38,6.03 32.38,2.38 D8.C | BOD_SW1.1 SW1.PIN_COM
XI  (via drill 0.7)
  Top 0.61: IC3.7 14.13,20.8 v15.24,21.91
  Bottom 0.813: C6.2 Q1.1
  Bottom 1.016: v15.24,21.91 17.46,21.91 17.46,26.35 C6.2
XO  (via drill 0.7)
  Top 0.61: IC3.8 v16.51,19.53
  Bottom 0.813: Q1.2 C7.1 19.21,21.27 19.21,19.53 v16.51,19.53
(copper drawn outside any net)
  shapes: Bottom circle x6, Top circle x6

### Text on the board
tPlace: G | B | C | D | G | V | C | D | I | V | G | Vin | S | D | GND | G | DAT | Micro SD / card | Vcc | SQM-BAS | GND | Ver: 2 | RK | Vcc | A | GK | DIO | BK | CLK | M | P | OK | C
bPlace: http://sqm.astromik.org | Vcc | Vcc | I2C-EXT | SDA | SCL | GND | EXT | ON | PWR | Vcc | B | A | GND
t_nam_doc: BAT1 / SC1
